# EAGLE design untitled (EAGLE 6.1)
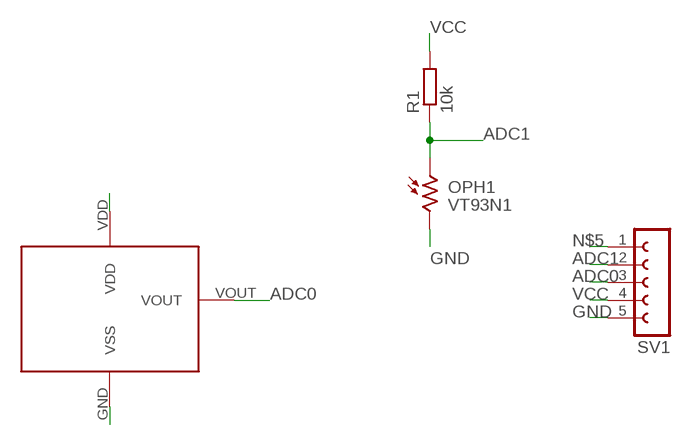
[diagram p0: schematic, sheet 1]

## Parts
OPH1  VT93N1  [VT900]
R1  10k  R-EU_0204/7  [0204/7]
SV1  FE05-1  [FE05-1]
U$1  LM35  [TO-92]

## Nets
ADC0: SV1.3 U$1.VOUT
ADC1: OPH1.1 R1.1 SV1.2
GND: OPH1.2 SV1.5 U$1.GND(VSS)
N$5: SV1.1
VCC: R1.2 SV1.4 U$1.VDD

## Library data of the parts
OPH1 = photo-elements:VT9: Photoconductive Cell VT900 Series
R1 = resistor:R-EU_: RESISTOR, European symbol
SV1 = con-lsta:FE05-1: FEMALE HEADER; OC_FARNELL: unknown; OC_NEWARK: unknown
U$1 = LM35:LM35

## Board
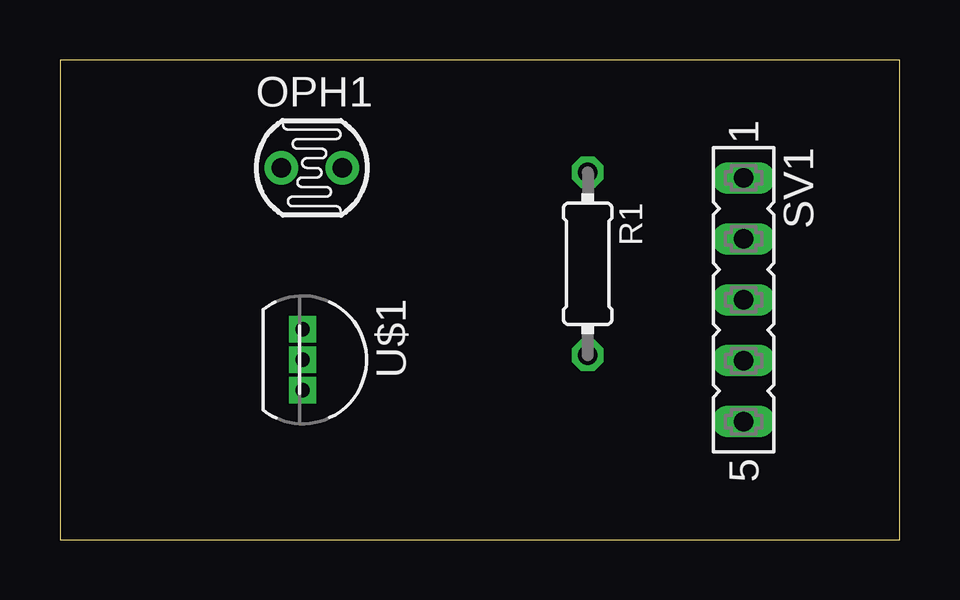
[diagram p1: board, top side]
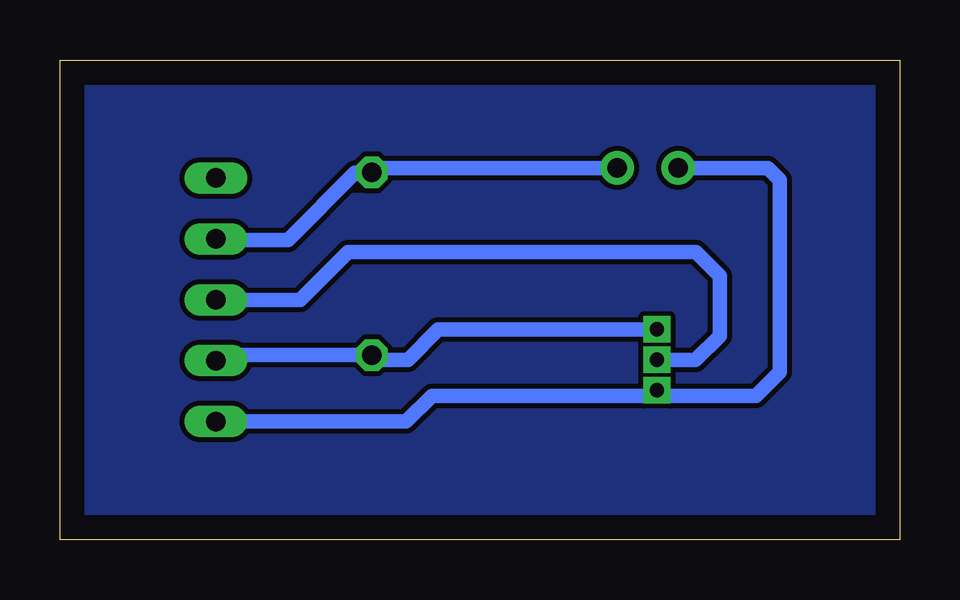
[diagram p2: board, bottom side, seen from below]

Size 35 x 20 mm. Coordinates in mm from the lower left corner, seen from the top.
Outline: 0,0 35,0 35,20 0,20 0,0
Copper layers (1*16): Top 0.035mm / dielectric 1.5mm / Bottom 0.035mm
Design rules: minimum track width 10mil, minimum drill 24mil, track to track 8mil, track to pad 8mil, pad to pad 8mil, via to via 8mil, smd to smd 8mil, copper to edge 40mil, drill to drill 8mil, minimum pad ring 10mil, minimum via ring 8mil, stop-mask expansion 4mil, vias tented up to drill 0mil, thermal gap 10mil

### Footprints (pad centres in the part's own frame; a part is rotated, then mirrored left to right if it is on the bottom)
VT900 = drill 0.8 pad 1.4: 1 -1.27,0; 2 1.27,0
0204/7 = drill 0.813 octagon: 1 -3.81,0; 2 3.81,0
FE05-1 = drill 0.813 long: 1 -5.08,0; 2 -2.54,0; 3 0,0; 4 2.54,0; 5 5.08,0
TO-92 = drill 0.6 square: GND 1.273,0.114; VDD -1.267,0.114; VOUT 0.003,0.114

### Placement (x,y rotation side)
OPH1  10.5,15.5 180 top
R1  22,11.5 270 top
SV1  28.5,10 270 top
U$1  10,7.5 270 top

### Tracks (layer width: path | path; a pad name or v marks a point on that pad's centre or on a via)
ADC0
  Bottom 0.61: U$1.VOUT 8.5,7.5 7.5,8.5 7.5,11 8.5,12 23,12 25,10 SV1.3
ADC1
  Bottom 0.61: OPH1.1 21.81,15.5 R1.1 22.69,15.31 25.5,12.5 28.46,12.5 SV1.2
GND
  Bottom 0.61: OPH1.2 5.5,15.5 5,15 5,7 6,6 9.89,6 U$1.GND 10.34,6 19.5,6 20.58,4.92 SV1.5
N$1
  pour Bottom: 0,20 0,0 35,0 35,20
VCC
  Bottom 0.61: SV1.4 28.27,7.69 R1.2 21.81,7.5 20.5,7.5 19.23,8.77 U$1.VDD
